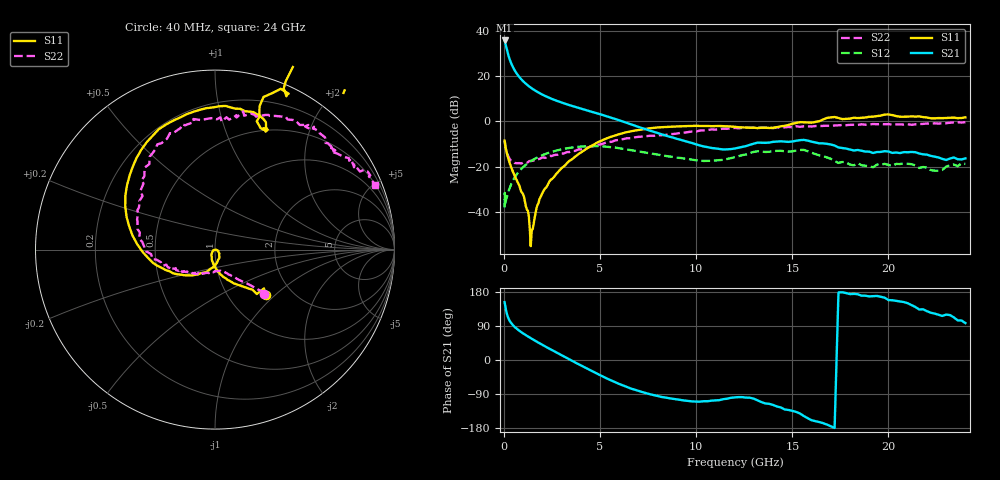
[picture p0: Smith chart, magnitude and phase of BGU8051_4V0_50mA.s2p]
! BGU8051_4V0_50mA
! Date/time Tue Jun 16 11:08:37 2015
! VAR V_out= 4.0000
! VAR I_out= 50.0100
! VAR V_in= 5.5450
! VAR I_in= 0.6879
# MHz S MA R 50
!  Freq-MHz  S11-mag  S11-arg  S21-mag  S21-arg  S12-mag  S12-arg  S22-mag  S22-arg
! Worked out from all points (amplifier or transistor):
!   187 points, 40 MHz to 24 GHz, reference 50 ohm
!   highest |S21| = 35.7 dB at 40 MHz (marker M1)
!   |S21| within 3 dB of that: start of sweep to 126.2 MHz
!   unconditionally stable (mu >= 1): 404.5 MHz to 13.27 GHz; 13.48 GHz to 14.01 GHz
!   at 750 MHz: K = 1.02, MAG = 20.5 dB, |S12| = -22.4 dB
!   at 5.4 GHz: K = 1.19, MAG = 4.0 dB, |S12| = -11.2 dB
!   at 24 GHz: K = -0.50, MSG = 1.2 dB, |S12| = -18.7 dB
!   lowest NFmin = 0.37 dB at 400 MHz
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40  0.3786 -41.8  60.96 152.6  0.01271 32.8  0.3706 -42.3
60  0.34 -46.7  56.71 146.6  0.02075 28.8  0.3268 -42.8
80  0.2906 -48.7  51.93 140.6  0.01645 39.9  0.2794 -45.2
120  0.2376 -56.4  44.23 130.0  0.01924 46.6  0.2337 -49.3
160  0.1997 -63.4  37.64 121.6  0.02172 50.3  0.2047 -52.9
200  0.1711 -69.4  32.41 115.2  0.02481 54.9  0.183 -56.5
260  0.1398 -78.3  26.59 107.7  0.03047 57.9  0.1608 -60.3
320  0.1148 -83.5  22.37 102.0  0.03587 59.9  0.1466 -63.6
400  0.09222 -91.3  18.36 96.2  0.04346 62.2  0.1359 -67.2
500  0.07416 -97.9  14.97 90.4  0.05254 62.5  0.1272 -73.0
700  0.04802 -111.9  10.9 81.3  0.07128 60.6  0.1204 -80.8
900  0.02878 -128.4  8.565 73.7  0.08956 57.9  0.1193 -89.7
1400  0.001793 -79.1  5.56 57.6  0.1335 48.6  0.1354 -107.2
1500  0.004232 -12.5  5.201 54.5  0.1418 46.5  0.1366 -109.3
2500  0.05388 -64.9  3.137 26.2  0.2151 24.6  0.1743 -131.5
4100  0.2197 -139.2  1.872 -16.8  0.2825 -11.7  0.2465 -154.5
6200  0.5554 154.2  0.995 -67.3  0.2508 -54.6  0.4079 173.9
8200  0.7491 111.0  0.523 -97.6  0.1804 -75.7  0.5008 147.3
12200  0.7478 67.7  0.2647 -97.9  0.1723 -75.2  0.7121 103.6
16200  0.9758 66.9  0.3453 -161.5  0.1913 -148.8  0.7926 70.5
20200  1.383 33.6  0.2032 157.7  0.1052 -154.3  0.8557 44.0
24000  1.234 20.9  0.1537 97.4  0.1161 -172.4  0.963 22.0
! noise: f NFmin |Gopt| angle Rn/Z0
400  0.3687  0.04559  360  0.0505
550  0.374  0.02214  18.89  0.0504
950  0.401  0.04123  154  0.05
1250  0.4334  0.07618  165.6  0.0496
1600  0.4845  0.1108  173.3  0.0495
1900  0.5397  0.1361  178.9  0.05
2250  0.6172  0.1621  185.4  0.0516
2600  0.7091  0.1859  191.8  0.0545
3300  0.9356  0.2326  204  0.066
4000  1.219  0.2839  214.5  0.0874
